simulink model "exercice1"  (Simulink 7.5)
settings: Solver=ode45  StartTime=0.0  StopTime=10.0  RelTol=1e-3

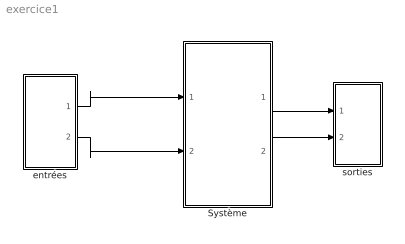
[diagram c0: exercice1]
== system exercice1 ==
  Système : Subsystem
  entrées : Subsystem
  sorties : Subsystem
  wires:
  entrées/1("u1 ") -> Système/1(u1)
  entrées/2("u2 ") -> Système/2(u2)
  Système/1("h ") -> sorties/1(h)
  Système/2("C ") -> sorties/2(C)

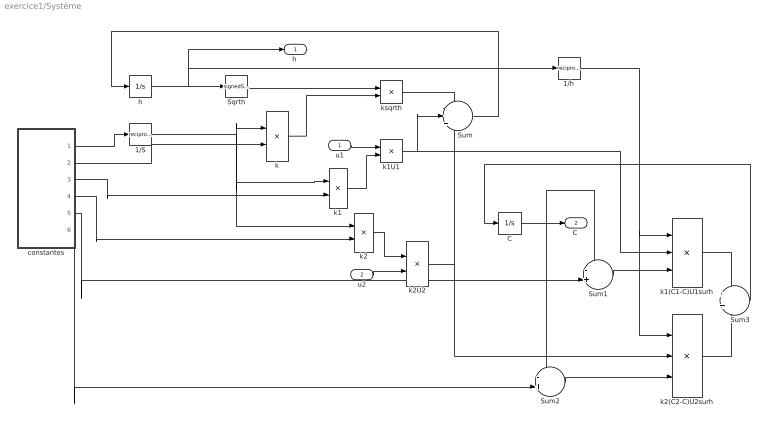
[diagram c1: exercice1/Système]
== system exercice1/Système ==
  u1 : Inport
  u2 : Inport  Port=2
  1/S : Math  Operator=reciprocal  OutDataType=fixdt(1, 16)  OutScaling=2^0
  1/h : Math  Operator=reciprocal  OutDataType=fixdt(1, 16)  OutScaling=2^0
  C : Integrator  InitialCondition=1
  Sqrth : Sqrt  Operator=signedSqrt
  Sum : Sum  Inputs=-++  OutDataType=fixdt(1, 16)  OutScaling=2^0
  Sum1 : Sum  Inputs=-+  OutDataType=fixdt(1, 16)  OutScaling=2^0
  Sum2 : Sum  Inputs=-+  OutDataType=fixdt(1, 16)  OutScaling=2^0
  Sum3 : Sum  OutDataType=fixdt(1, 16)  OutScaling=2^0
  constantes : Subsystem
  h : Integrator  InitialCondition=1
  k : Product  OutDataType=fixdt(1, 16)  OutScaling=2^0
  k1 : Product  OutDataType=fixdt(1, 16)  OutScaling=2^0
  k1(C1-C)U1surh : Product  Inputs=3  OutDataType=fixdt(1, 16)  OutScaling=2^0
  k1U1 : Product  OutDataType=fixdt(1, 16)  OutScaling=2^0
  k2 : Product  OutDataType=fixdt(1, 16)  OutScaling=2^0
  k2(C2-C)U2surh : Product  Inputs=3  OutDataType=fixdt(1, 16)  OutScaling=2^0
  k2U2 : Product  OutDataType=fixdt(1, 16)  OutScaling=2^0
  ksqrth : Product  OutDataType=fixdt(1, 16)  OutScaling=2^0
  "h " : Outport
  "C " : Outport  Port=2
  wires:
  constantes/1("S ") -> 1/S/1
  constantes/2("alpha ") -> k/2
  1/S/1 -> k/1, k1/1, k2/1
  constantes/3("alpha1 ") -> k1/2
  constantes/4("alpha2 ") -> k2/2
  k1/1 -> k1U1/2
  k2/1 -> k2U2/1
  h/1 -> Sqrth/1, 1/h/1, "h "/1
  k/1 -> ksqrth/2
  Sqrth/1 -> ksqrth/1
  ksqrth/1 -> Sum/1
  k1U1/1 -> Sum/2, k1(C1-C)U1surh/2
  k2U2/1 -> Sum/3, k2(C2-C)U2surh/2
  Sum/1 -> h/1
  constantes/5("C1  ") -> Sum1/2
  C/1 -> Sum1/1, Sum2/1, "C "/1
  constantes/6("C2 ") -> Sum2/2
  Sum1/1 -> k1(C1-C)U1surh/3
  k1(C1-C)U1surh/1 -> Sum3/1
  k2(C2-C)U2surh/1 -> Sum3/2
  Sum3/1 -> C/1
  1/h/1 -> k2(C2-C)U2surh/1, k1(C1-C)U1surh/1
  Sum2/1 -> k2(C2-C)U2surh/3
  u1/1 -> k1U1/1
  u2/1 -> k2U2/2

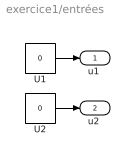
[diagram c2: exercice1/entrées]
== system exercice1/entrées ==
  U1 : Constant  Value=0  OutDataType=fixdt(1, 16)  OutScaling=2^0
  U2 : Constant  Value=0  OutDataType=fixdt(1, 16)  OutScaling=2^0
  "u1 " : Outport
  "u2 " : Outport  Port=2
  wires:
  U1/1 -> "u1 "/1
  U2/1 -> "u2 "/1

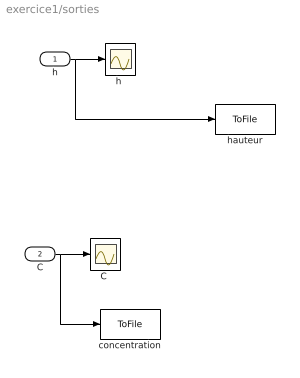
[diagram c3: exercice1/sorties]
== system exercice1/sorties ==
  h : Inport
  C : Inport  Port=2
  "C " : Scope
  concentration : ToFile  Filename=seri6C
  "h " : Scope
  hauteur : ToFile  Filename=seri6h
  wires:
  h/1 -> "h "/1, hauteur/1
  C/1 -> "C "/1, concentration/1

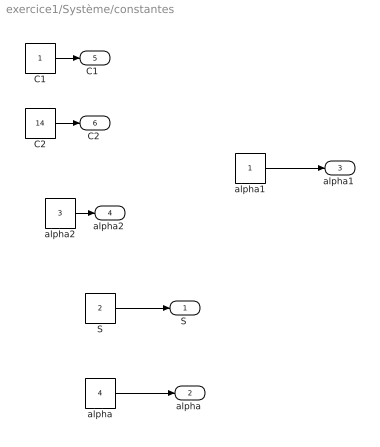
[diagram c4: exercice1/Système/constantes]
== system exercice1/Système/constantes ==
  C1 : Constant  OutDataType=fixdt(1, 16)  OutScaling=2^0
  C2 : Constant  Value=14  OutDataType=fixdt(1, 16)  OutScaling=2^0
  S : Constant  Value=2  OutDataType=fixdt(1, 16)  OutScaling=2^0
  alpha : Constant  Value=4  OutDataType=fixdt(1, 16)  OutScaling=2^0
  alpha1 : Constant  OutDataType=fixdt(1, 16)  OutScaling=2^0
  alpha2 : Constant  Value=3  OutDataType=fixdt(1, 16)  OutScaling=2^0
  "S " : Outport
  "alpha " : Outport  Port=2
  "alpha1 " : Outport  Port=3
  "alpha2 " : Outport  Port=4
  "C1  " : Outport  Port=5
  "C2 " : Outport  Port=6
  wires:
  C1/1 -> "C1  "/1
  C2/1 -> "C2 "/1
  alpha2/1 -> "alpha2 "/1
  S/1 -> "S "/1
  alpha1/1 -> "alpha1 "/1
  alpha/1 -> "alpha "/1
